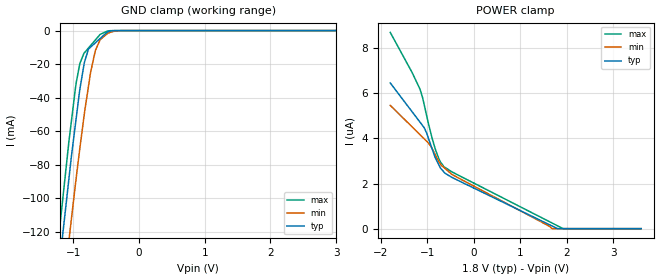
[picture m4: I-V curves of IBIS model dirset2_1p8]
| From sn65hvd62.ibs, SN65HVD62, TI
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|   dirset2_1p8 Model
[Model]   dirset2_1p8
Model_type   Input
Vinl = 0.54
Vinh = 1.26
|   typ   min   max
|   (nom PVT)   (fast PVT)   (slow PVT)
 C_comp   1.444e-12   1.437e-12   1.465e-12
| Where nom  PVT is Nominal Process, 1.8V, 27C
|   Fast PVT is Strong Process,  1.98V, -40C
|   Slow PVT is Weak Process,   1.62V, 125C
[Voltage Range]   1.8   1.62   1.98
|Ambient Temperature   25   85   -40
|Junction Temperature
[Temperature Range]   27   125   -40
[Power Clamp Reference]   1.8   1.62   1.98
[GND Clamp Reference]   0   0   0
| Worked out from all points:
|   GND clamp passes 1 mA (typ) near -0.49 V on its own axis
[GND Clamp]
|   Voltage   I(typ)   I(min)   I(max)
-1.8V     -363.3mA   -388.4mA   -351.2mA
-1.224V   -143.9mA   -180mA     -123.7mA
-1.158V   -120.4mA   -155.9mA   -99.39mA
-1.068V   -88.62mA   -125.5mA   -66.41mA
-1.031V   -75.86mA   -113.2mA   -54.83mA
-954.2mV  -51.76mA   -87.32mA   -30.78mA
-900.5mV  -35.02mA   -70.24mA   -19.66mA
-831.6mV  -19.03mA   -49.53mA   -13.28mA
-737.5mV  -9.866mA   -25.09mA   -8.966mA
-591.4mV  -4.706mA   -5.384mA   -2.256mA
-285.6mV  -7.004uA   -69.45uA   -1.314uA
3.6V      0A         0A         0A
[POWER Clamp]
|   Voltage   I(typ)   I(min)   I(max)
-1.8V     6.465uA    5.47uA     8.706uA
-1.162V   4.73uA     4.174uA    6.197uA
-1.104V   4.574uA    4.057uA    5.817uA
-1.015V   4.239uA    3.876uA    5.002uA
-919mV    3.659uA    3.633uA    4.177uA
-823.7mV  3.122uA    3.251uA    3.486uA
-720mV    2.692uA    2.866uA    2.961uA
-649mV    2.522uA    2.719uA    2.755uA
-478.8mV  2.28uA     2.416uA    2.525uA
1.678V    121.8nA    0A         254.3nA
1.918V    0A         0A         0A
3.6V      0A         0A         0A
